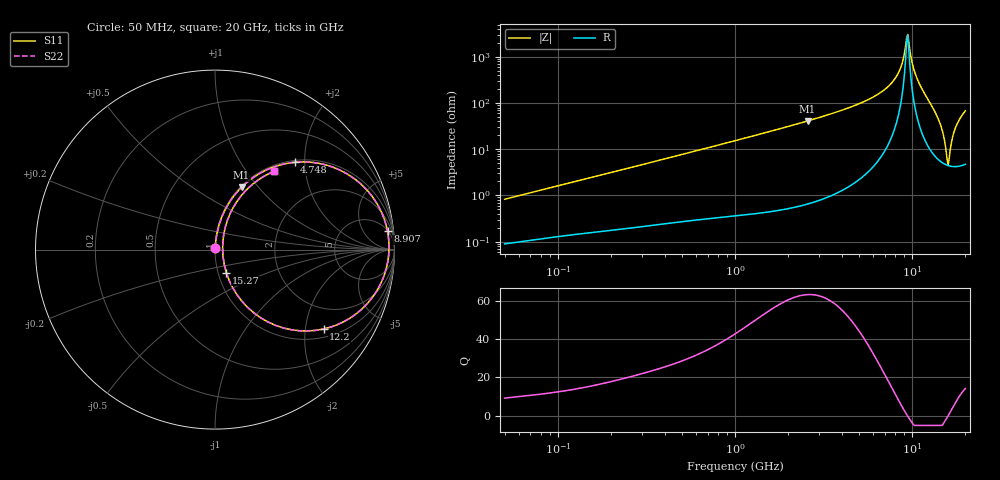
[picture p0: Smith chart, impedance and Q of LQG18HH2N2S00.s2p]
!Murata Part Number: LQG18HH2N2S00
!These Parameters are Measured in Series Mode Connection
!  o--[Z]--o
!Port1  Port2
!  o-------o
!Freq. Start=50[MHz] Stop=20[GHz], 401[Steps]
# Hz S RI R 50
!Freq.(Hz) S11(Real) S11(Imag) S21(Real) S21(Imag) S12(Real) S12(Imag) S22(Real) S22(Imag)
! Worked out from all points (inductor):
!   401 points, 50 MHz to 20 GHz, reference 50 ohm
!   read as one part in series: L = 2.59 nH near 51.52 MHz
!   highest Q = 63.2 at 2.569 GHz (marker M1), where L = 2.54 nH
!   self-resonance near 9.317 GHz
!   S11 on the Smith chart (normalised r, x): 50 MHz: 1.00, +0.02; 4.748 GHz: 1.04, +1.78; 8.907 GHz: 6, +17; 12.2 GHz: 1.25, -2.51; 15.27 GHz: 1.10, -0.29; 20 GHz: 1.09, +1.36
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5e7  0.000953 0.00819  0.999 -0.00819  0.999 -0.00819  0.000953 0.00819
1.364002e8  0.00194 0.0215  0.9981 -0.0215  0.9981 -0.0215  0.00194 0.0215
3.721004e8  0.00559 0.0569  0.9944 -0.0569  0.9944 -0.0569  0.00559 0.0569
1e9  0.0262 0.1484  0.9738 -0.1484  0.9738 -0.1484  0.0262 0.1484
2.569357e9  0.148 0.3473  0.852 -0.3473  0.852 -0.3473  0.148 0.3473
2.728004e9  0.1654 0.3637  0.8346 -0.3637  0.8346 -0.3637  0.1654 0.3637
4.748272e9  0.443 0.4863  0.557 -0.4863  0.557 -0.4863  0.443 0.4863
7.442007e9  0.8406 0.3378  0.1594 -0.3378  0.1594 -0.3378  0.8406 0.3378
8.264682e9  0.9235 0.2168  0.0765 -0.2168  0.0765 -0.2168  0.9235 0.2168
8.907419e9  0.9612 0.1018  0.0388 -0.1018  0.0388 -0.1018  0.9612 0.1018
9.178299e9  0.9682 0.0492  0.0318 -0.0492  0.0318 -0.0492  0.9682 0.0492
9.457416e9  0.9692 -0.00657  0.0308 0.00657  0.0308 0.00657  0.9692 -0.00657
1.050288e10  0.9092 -0.2167  0.0908 0.2167  0.0908 0.2167  0.9092 -0.2167
1.220001e10  0.6046 -0.4425  0.3954 0.4425  0.3954 0.4425  0.6046 -0.4425
1.396067e10  0.2167 -0.353  0.7833 0.353  0.7833 0.353  0.2167 -0.353
1.460232e10  0.1219 -0.2507  0.8781 0.2507  0.8781 0.2507  0.1219 -0.2507
1.527346e10  0.0629 -0.1276  0.9371 0.1276  0.9371 0.1276  0.0629 -0.1276
1.573793e10  0.0451 -0.041  0.9549 0.041  0.9549 0.041  0.0451 -0.041
1.621653e10  0.0438 0.0446  0.9562 -0.0446  0.9562 -0.0446  0.0438 0.0446
1.696185e10  0.0694 0.1641  0.9306 -0.1641  0.9306 -0.1641  0.0694 0.1641
1.774144e10  0.1212 0.2665  0.8788 -0.2665  0.8788 -0.2665  0.1212 0.2665
2e10  0.3271 0.4354  0.6729 -0.4354  0.6729 -0.4354  0.3271 0.4354
